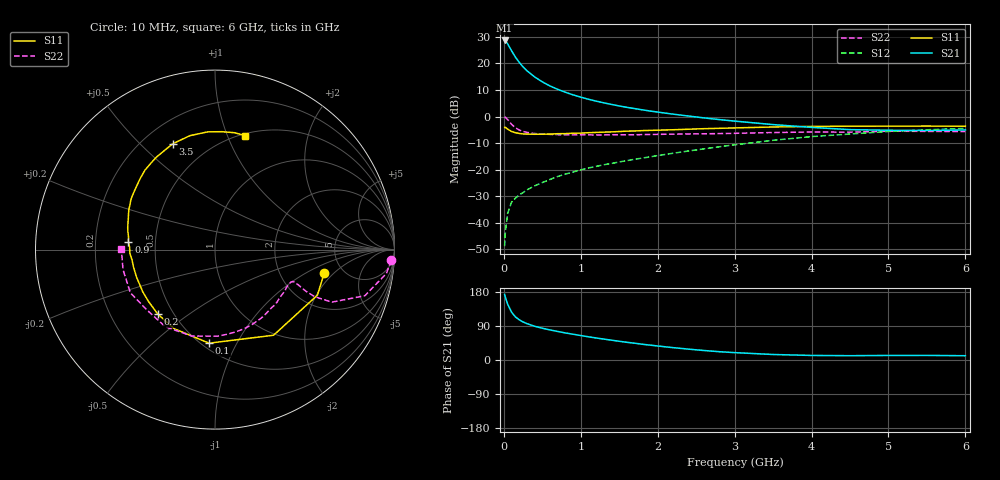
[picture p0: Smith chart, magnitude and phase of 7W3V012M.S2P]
! Infineon Technologies  Discrete & RF Semiconductors
! BFS17W
! Si NPN RF Bipolar Junction Transistor in SOT323
! VCE = 3 V  IC = 12 mA
! Common Emitter S-Parameters:  August  1999
# GHz  S  MA  R  50
!  f  S11  S21  S12  S22
! GHz  MAG  ANG  MAG  ANG  MAG  ANG  MAG  ANG
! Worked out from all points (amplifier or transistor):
!   36 points, 10 MHz to 6 GHz, reference 50 ohm
!   highest |S21| = 28.7 dB at 10 MHz (marker M1)
!   |S21| within 3 dB of that: start of sweep to 83.15 MHz
!   unconditionally stable (mu >= 1): 362.8 MHz to 2.503 GHz; 4.429 GHz to end of sweep
!   at 250 MHz: K = 0.86, MSG = 23.7 dB, |S12| = -28.7 dB
!   at 1.4 GHz: K = 1.21, MAG = 8.4 dB, |S12| = -17.7 dB
!   at 6 GHz: K = 1.07, MAG = -1.9 dB, |S12| = -4.5 dB
!   S11 on the Smith chart (normalised r, x): 10 MHz: 3.62, -1.52; 100 MHz: 0.54, -0.78; 200 MHz: 0.41, -0.38; 900 MHz: 0.35, +0.04; 3.5 GHz: 0.32, +0.63; 6 GHz: 0.52, +1.16
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0.01  0.6229 -11.9  27.15 173.1  0.0036 82.7  0.9836 -3.5
0.02  0.6244 -24.0  26.73 165.6  0.0068 81.8  0.9644 -7.9
0.05  0.5781 -55.6  23.42 147.0  0.015 69.4  0.8738 -17.1
0.1  0.5224 -93.6  17.38 126.4  0.0243 57.6  0.714 -24.2
0.15  0.4959 -117.3  13.2 113.9  0.0288 53.6  0.6138 -25.3
0.2  0.4801 -131.7  10.49 106.1  0.0333 54.4  0.5572 -24.6
0.25  0.4698 -142.1  8.618 100.4  0.0368 55.1  0.5225 -23.6
0.3  0.4663 -149.5  7.297 96.0  0.0414 56.9  0.5025 -22.9
0.4  0.4632 -160.4  5.576 89.1  0.0493 60.1  0.4777 -22.3
0.5  0.4643 -167.5  4.504 83.9  0.0569 61.9  0.4669 -22.4
0.6  0.4658 -172.9  3.764 79.3  0.0652 63.9  0.4604 -23.2
0.7  0.4745 -177.4  3.259 75.3  0.0741 65.1  0.4556 -24.6
0.9  0.4841 175.1  2.559 68.0  0.0899 66.1  0.4502 -28.1
1.1  0.4954 168.4  2.118 61.2  0.1072 66.9  0.4506 -32.6
1.3  0.5081 162.5  1.81 55.1  0.1233 67.4  0.4497 -37.7
1.6  0.5304 154.8  1.488 46.7  0.1475 67.8  0.4518 -45.6
2.2  0.563 140.6  1.109 32.6  0.2031 68.1  0.4655 -63.4
2.8  0.5991 126.8  0.876 21.9  0.2687 65.8  0.4768 -82.3
3.5  0.6349 111.8  0.704 14.5  0.3567 60.1  0.4987 -105.0
4.5  0.6573 93.5  0.566 11.4  0.468 47.5  0.507 -138.7
5.5  0.6603 80.4  0.544 12.1  0.5616 35.0  0.5245 -167.8
6  0.6562 75.3  0.558 11.3  0.5982 28.9  0.5216 179.5
